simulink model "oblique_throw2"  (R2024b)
settings: Solver=VariableStepAuto  StartTime=0.0  StopTime=3  RelTol=1e-3
libraries: simulink x2

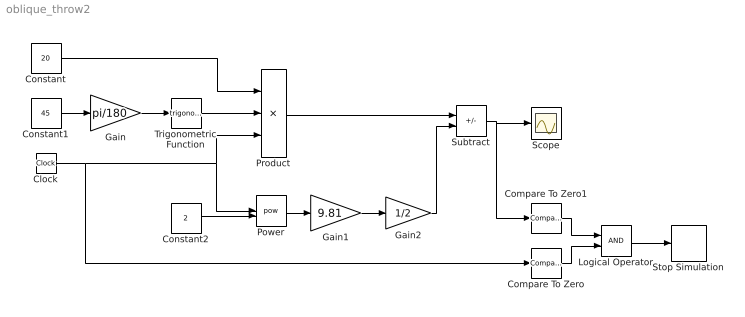
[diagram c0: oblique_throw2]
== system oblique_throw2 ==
  Clock : Clock
  Compare To Zero : simulink/Logic and Bit Operations/Compare To Zero  relop=>  OutDataTypeStr=boolean
  Compare To Zero1 : simulink/Logic and Bit Operations/Compare To Zero  relop=<=  OutDataTypeStr=boolean
  Constant : Constant  Value=20
  Constant1 : Constant  Value=45
  Constant2 : Constant  Value=2
  Gain : Gain  Gain=pi/180
  Gain1 : Gain  Gain=9.81
  Gain2 : Gain  Gain=1/2
  Logical Operator : Logic  AllPortsSameDT=off  OutDataTypeStr=boolean
  Power : Math  Operator=pow
  Product : Product  Inputs=3
  Scope : Scope
  Stop Simulation : Stop
  Subtract : Sum  Inputs=+-
  Trigonometric Function : Trigonometry
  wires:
  Constant1/1 -> Gain/1
  Gain/1 -> Trigonometric Function/1
  Trigonometric Function/1 -> Product/2
  Clock/1 -> Product/3, Power/1, Compare To Zero/1
  Constant/1 -> Product/1
  Constant2/1 -> Power/2
  Power/1 -> Gain1/1
  Gain1/1 -> Gain2/1
  Product/1 -> Subtract/1
  Gain2/1 -> Subtract/2
  Subtract/1 -> Compare To Zero1/1, Scope/1
  Compare To Zero1/1 -> Logical Operator/1
  Compare To Zero/1 -> Logical Operator/2
  Logical Operator/1 -> Stop Simulation/1
